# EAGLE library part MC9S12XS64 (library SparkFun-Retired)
Freescale 16-bit uC Dead prototype
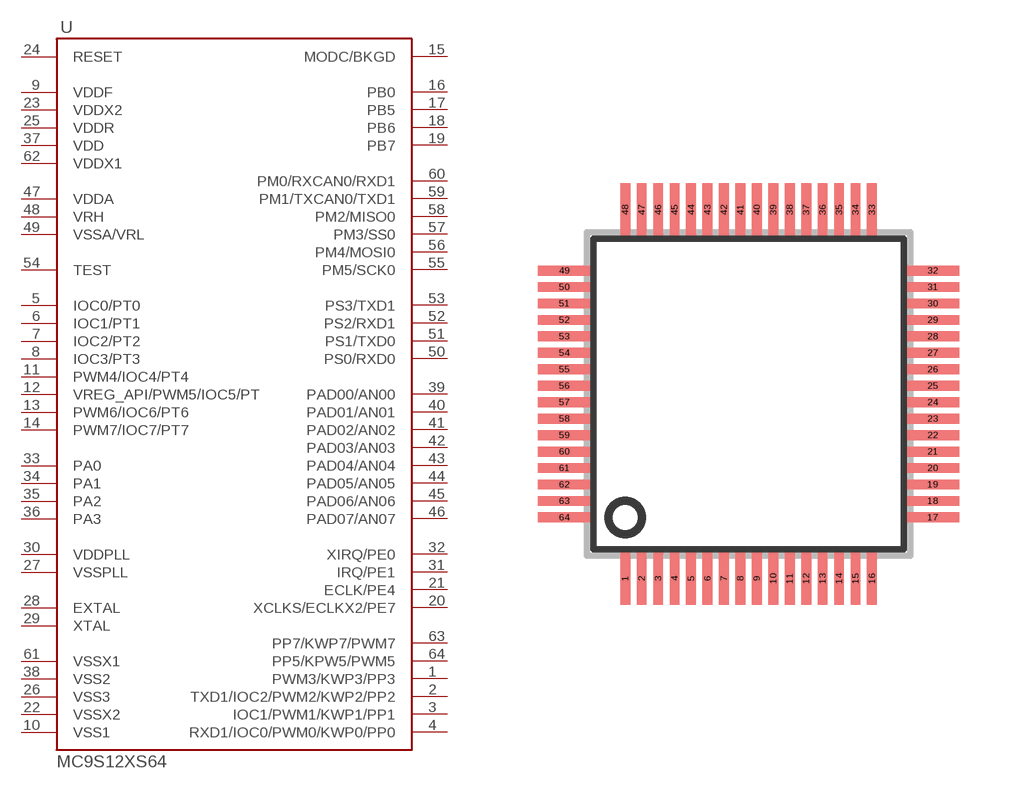
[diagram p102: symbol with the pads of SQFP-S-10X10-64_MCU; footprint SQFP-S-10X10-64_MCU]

Designator prefix -

## MC9S12XS64 (PROD_ID: IC-09432; VALUE: MC9S12XS64)  [SQFP-S-10X10-64_MCU]
1  PWM3/KWP3/PP3
2  TXD1/IOC2/PWM2/KWP2/PP2
3  IOC1/PWM1/KWP1/PP1
4  RXD1/IOC0/PWM0/KWP0/PP0
5  IOC0/PT0
6  IOC1/PT1
7  IOC2/PT2
8  IOC3/PT3
9  VDDF
10  VSS1
11  PWM4/IOC4/PT4
12  VREG_API/PWM5/IOC5/PT
13  PWM6/IOC6/PT6
14  PWM7/IOC7/PT7
15  MODC/BKGD
16  PB0
17  PB5
18  PB6
19  PB7
20  XCLKS/ECLKX2/PE7
21  ECLK/PE4
22  VSSX2
23  VDDX2
24  RESET
25  VDDR
26  VSS3
27  VSSPLL
28  EXTAL
29  XTAL
30  VDDPLL
31  IRQ/PE1
32  XIRQ/PE0
33  PA0
34  PA1
35  PA2
36  PA3
37  VDD
38  VSS2
39  PAD00/AN00
40  PAD01/AN01
41  PAD02/AN02
42  PAD03/AN03
43  PAD04/AN04
44  PAD05/AN05
45  PAD06/AN06
46  PAD07/AN07
47  VDDA
48  VRH
49  VSSA/VRL
50  PS0/RXD0
51  PS1/TXD0
52  PS2/RXD1
53  PS3/TXD1
54  TEST
55  PM5/SCK0
56  PM4/MOSI0
57  PM3/SS0
58  PM2/MISO0
59  PM1/TXCAN0/TXD1
60  PM0/RXCAN0/RXD1
61  VSSX1
62  VDDX1
63  PP7/KWP7/PWM7
64  PP5/KPW5/PWM5

## Footprint SQFP-S-10X10-64_MCU (pad centres in mm)
QFP64 shrink quad flat pack, square
smd 0.3 x 1.6: 1 -3.75,-5.6; 2 -3.25,-5.6; 3 -2.75,-5.6; 4 -2.25,-5.6; 5 -1.75,-5.6; 6 -1.25,-5.6; 7 -0.75,-5.6; 8 -0.25,-5.6; 9 0.25,-5.6; 10 0.75,-5.6; 11 1.25,-5.6; 12 1.75,-5.6; 13 2.25,-5.6; 14 2.75,-5.6; 15 3.25,-5.6; 16 3.75,-5.6; 33 3.75,5.6; 34 3.25,5.6; 35 2.75,5.6; 36 2.25,5.6; 37 1.75,5.6; 38 1.25,5.6; 39 0.75,5.6; 40 0.25,5.6; 41 -0.25,5.6; 42 -0.75,5.6; 43 -1.25,5.6; 44 -1.75,5.6; 45 -2.25,5.6; 46 -2.75,5.6; 47 -3.25,5.6; 48 -3.75,5.6
smd 1.6 x 0.3: 17 5.6,-3.75; 18 5.6,-3.25; 19 5.6,-2.75; 20 5.6,-2.25; 21 5.6,-1.75; 22 5.6,-1.25; 23 5.6,-0.75; 24 5.6,-0.25; 25 5.6,0.25; 26 5.6,0.75; 27 5.6,1.25; 28 5.6,1.75; 29 5.6,2.25; 30 5.6,2.75; 31 5.6,3.25; 32 5.6,3.75; 49 -5.6,3.75; 50 -5.6,3.25; 51 -5.6,2.75; 52 -5.6,2.25; 53 -5.6,1.75; 54 -5.6,1.25; 55 -5.6,0.75; 56 -5.6,0.25; 57 -5.6,-0.25; 58 -5.6,-0.75; 59 -5.6,-1.25; 60 -5.6,-1.75; 61 -5.6,-2.25; 62 -5.6,-2.75; 63 -5.6,-3.25; 64 -5.6,-3.75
